(* Logix 5000 AddOnInstructionDefinition export NXEE2_Generic_ch2_setup; software revision 20.03 *)

ADD_ON_INSTRUCTION NXEE2_Generic_ch2_setup   (* revision 1.0, ExecuteEnableInFalse *)
// Revision note:
// Revision 1.0: 4/6/2021 initial release
VAR_INPUT
   Ch1_Status_Word : INT; {required}
        .4   // command error
        .5   // config error
        .6   // sutup error
        .7   // scalars errors
        .8   // preset value error
        .9   // full scale count error
        .15   // ACK bit
   Ch2_Status_Word : INT; {required}
        .4   // command error
        .5   // config error
        .6   // setup error
        .7   // scalar errors
        .8   // preset value error
        .9   // full scale count error
   Network_input_data_format : INT; {required}
   Input_function : INT; {required}
   data_logic_0_positive_1_negative : BOOL; {required}
   data_type_0_binary_1_gray_code : BOOL; {required}
   count_direction_0_normal_1_reverse : BOOL; {required}
   velocity_update_0_160ms_1_24ms : BOOL; {required}
   SSI_Clock_Frequency : INT; {required}
   LED_0_enable_1_disable : BOOL; {required}
   Swap_32_bit_words_endian_0_NO_1_YES : BOOL; {required}
   save_in_flash_0_NO_1_YES : BOOL; {required}
   Number_of_SSI_Clock_Bits : INT; {required}
   MSB_Number : INT; {required}
   Number_of_Data_Bits : INT; {required}
   Scalar_Multiplier : INT; {required}
   Scalar_Divisor : INT; {required}
   Preset_Value : DINT; {required}
   Full_Scale_Count : DINT; {required}
END_VAR
VAR_OUTPUT
   EN : BOOL; {access Read Only, visible}
   DN : BOOL; {access Read Only, visible}
   ER : BOOL; {access Read Only, visible}
END_VAR
VAR_IN_OUT
   AMCI_NXEE2_output_data : INT[10]; {required}
END_VAR
VAR
   allow_programming : BOOL;
   command_data_block : INT[10];
        [0].0   // program channel 1
        [0].1   // program channel 2
        [0].2   // program ch0
        [0].4   // change channel 1 display format
        [0].5   // change channel 2 display format
        [0].14   // save to flash
        [0].15   // transmit bit
   internal_preset_value : DINT; {access None}
END_VAR

ROUTINE EnableInFalse   (* ladder *)
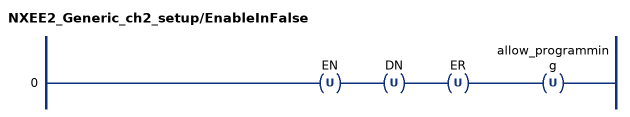
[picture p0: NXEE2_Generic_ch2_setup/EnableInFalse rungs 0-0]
   0: OTU(EN)OTU(DN)OTU(ER)OTU(allow_programming);
END_ROUTINE

ROUTINE Logic   (* ladder *)
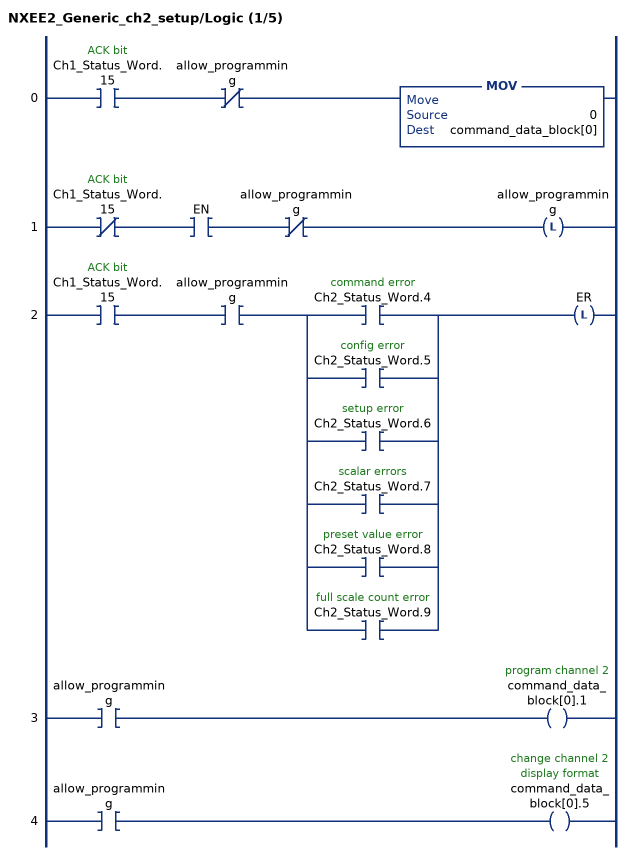
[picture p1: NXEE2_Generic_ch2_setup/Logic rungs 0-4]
   0: XIC(Ch1_Status_Word.15)XIO(allow_programming)MOV(0,command_data_block[0]);
   1: XIO(Ch1_Status_Word.15)XIC(EN)XIO(allow_programming)OTL(allow_programming);
   2: XIC(Ch1_Status_Word.15)XIC(allow_programming)[XIC(Ch2_Status_Word.4) ,XIC(Ch2_Status_Word.5) ,XIC(Ch2_Status_Word.6) ,XIC(Ch2_Status_Word.7) ,XIC(Ch2_Status_Word.8) ,XIC(Ch2_Status_Word.9) ]OTL(ER);
   3: XIC(allow_programming)OTE(command_data_block[0].1);
   4: XIC(allow_programming)OTE(command_data_block[0].5);
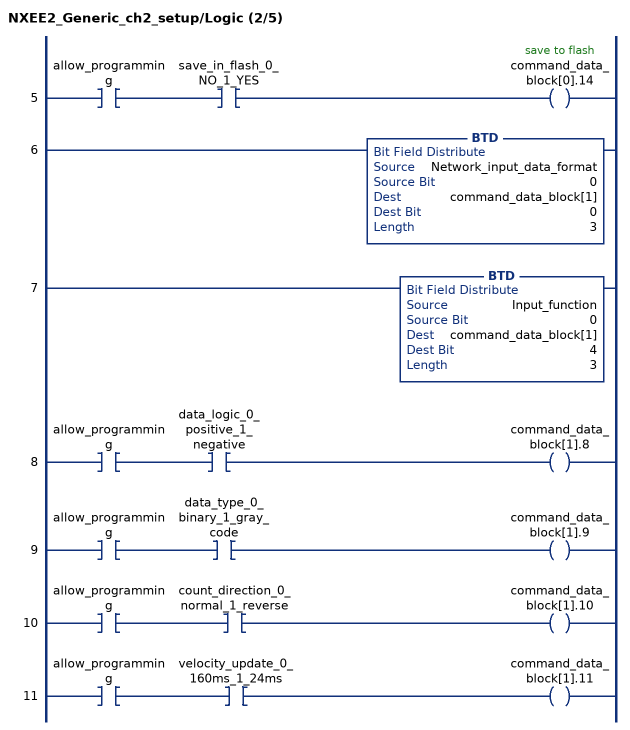
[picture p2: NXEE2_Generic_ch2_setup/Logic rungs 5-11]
   5: XIC(allow_programming)XIC(save_in_flash_0_NO_1_YES)OTE(command_data_block[0].14);
   6: BTD(Network_input_data_format,0,command_data_block[1],0,3);
   7: BTD(Input_function,0,command_data_block[1],4,3);
   8: XIC(allow_programming)XIC(data_logic_0_positive_1_negative)OTE(command_data_block[1].8);
   9: XIC(allow_programming)XIC(data_type_0_binary_1_gray_code)OTE(command_data_block[1].9);
   10: XIC(allow_programming)XIC(count_direction_0_normal_1_reverse)OTE(command_data_block[1].10);
   11: XIC(allow_programming)XIC(velocity_update_0_160ms_1_24ms)OTE(command_data_block[1].11);
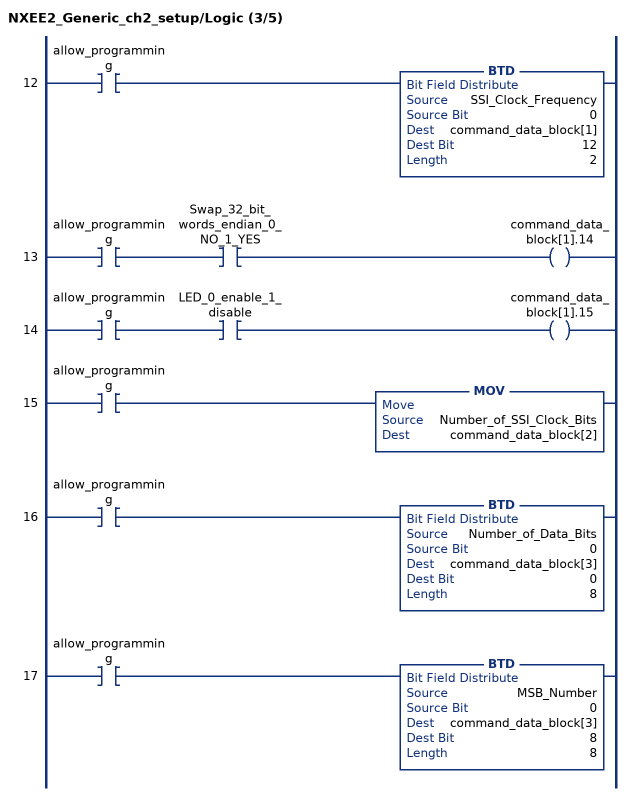
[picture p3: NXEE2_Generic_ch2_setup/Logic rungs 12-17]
   12: XIC(allow_programming)BTD(SSI_Clock_Frequency,0,command_data_block[1],12,2);
   13: XIC(allow_programming)XIC(Swap_32_bit_words_endian_0_NO_1_YES)OTE(command_data_block[1].14);
   14: XIC(allow_programming)XIC(LED_0_enable_1_disable)OTE(command_data_block[1].15);
   15: XIC(allow_programming)MOV(Number_of_SSI_Clock_Bits,command_data_block[2]);
   16: XIC(allow_programming)BTD(Number_of_Data_Bits,0,command_data_block[3],0,8);
   17: XIC(allow_programming)BTD(MSB_Number,0,command_data_block[3],8,8);
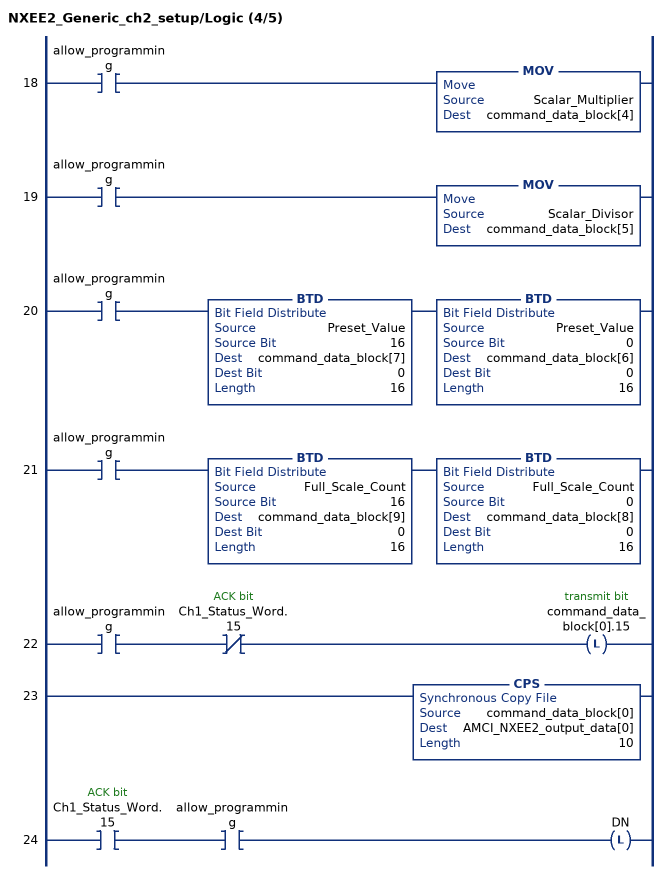
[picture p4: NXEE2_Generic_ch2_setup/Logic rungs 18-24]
   18: XIC(allow_programming)MOV(Scalar_Multiplier,command_data_block[4]);
   19: XIC(allow_programming)MOV(Scalar_Divisor,command_data_block[5]);
   20: XIC(allow_programming)BTD(Preset_Value,16,command_data_block[7],0,16)BTD(Preset_Value,0,command_data_block[6],0,16);
   21: XIC(allow_programming)BTD(Full_Scale_Count,16,command_data_block[9],0,16)BTD(Full_Scale_Count,0,command_data_block[8],0,16);
   22: XIC(allow_programming)XIO(Ch1_Status_Word.15)OTL(command_data_block[0].15);
   23: CPS(command_data_block[0],AMCI_NXEE2_output_data[0],10);
   24: XIC(Ch1_Status_Word.15)XIC(allow_programming)OTL(DN);
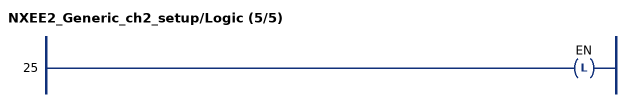
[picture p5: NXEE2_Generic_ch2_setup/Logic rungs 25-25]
   25: OTL(EN);
END_ROUTINE
END_ADD_ON_INSTRUCTION
